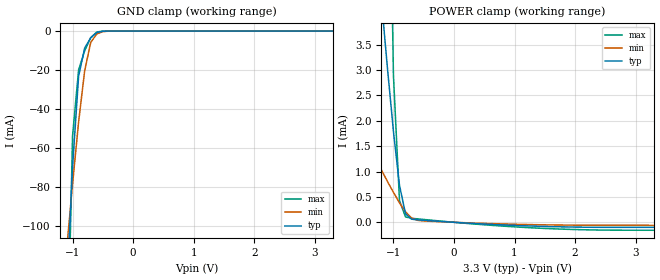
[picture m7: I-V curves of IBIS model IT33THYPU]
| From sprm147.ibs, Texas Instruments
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[Model]   IT33THYPU
Model_type   Input
Polarity   Non-Inverting
| signals   A, Y
Vinl = 0.8V
Vinh = 2.0V
|   typ   min   max
C_comp   0.89934336p   0.87230502p   0.9266069p
|   typ   min   max
[Temperature Range]   25   -40   125
|   typ   min   max
[Voltage Range]   3.30V   3.00V   3.60V
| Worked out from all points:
|   GND clamp passes 1 mA (typ) near -0.61 V on its own axis
|   POWER clamp passes 1 mA (typ) near -0.93 V on its own axis
[GND_clamp]
|   Voltage   I(typ)   I(min)   I(max)
-3.3V     -1.933A    -959mA     -4.949A
-1.1V     -136.4mA   -113mA     -192.6mA
-1V       -69.59mA   -78.55mA   -53.78mA
-900mV    -23.17mA   -46.64mA   -19.88mA
-800mV    -8.735mA   -20.39mA   -10.13mA
-700mV    -3.437mA   -5.826mA   -3.396mA
-600mV    -755.6uA   -1.47mA    -483.1uA
-500mV    -77.66uA   -274uA     -28.67uA
-400mV    -4.875uA   -34.93uA   -866.3nA
3.3V      222pA      20.56nA    0A
[POWER_clamp]
|   Voltage   I(typ)   I(min)   I(max)
-3.3V     35.07mA    6.127mA    227.3mA
-2.4V     21.74mA    3.905mA    136.5mA
-2.3V     20.26mA    3.661mA    126.5mA
-1.2V     4.393mA    1.033mA    18.59mA
-1.1V     3.053mA    807.6uA    9.9mA
-1V       1.793mA    589.5uA    2.902mA
-900mV    729.4uA    384.3uA    426.2uA
-800mV    164.6uA    205.2uA    105.2uA
-700mV    61.7uA     83.12uA    79.26uA
-500mV    39.14uA    26.17uA    55.9uA
1.3V      -74.37uA   -46.08uA   -109.7uA
3.3V      -100.1uA   -61.52uA   -157uA
